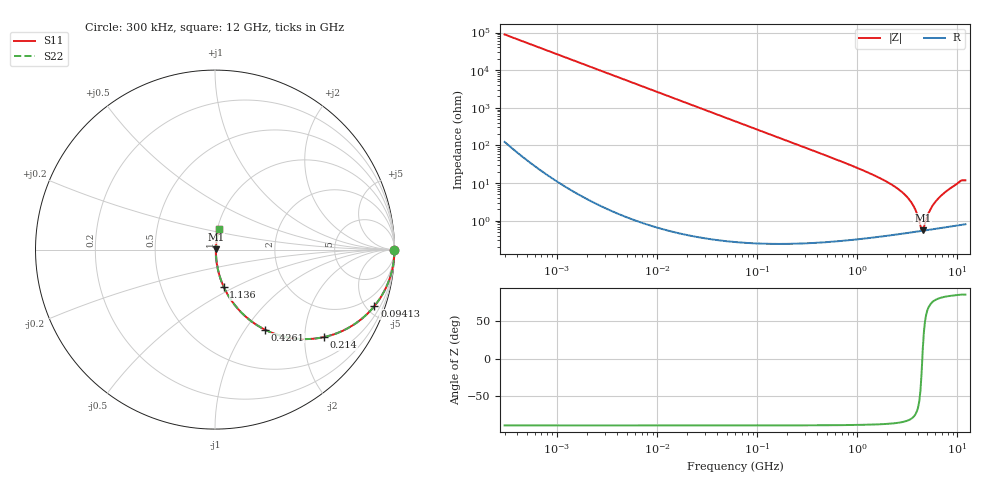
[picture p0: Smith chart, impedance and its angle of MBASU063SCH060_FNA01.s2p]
! MBASU063SCH060_FNA01  S-PARAMETER MODEL  ( Standard Model )
! Model Generated by TAIYO YUDEN Corporation (http://www.ty-top.com)
! Version 1.0
! TAIYO YUDEN Control No. 230609
! Copyright(c) 2023 TAIYO YUDEN CO.,LTD. All Rights Reserved.
! Product Description (link to TY-COMPAS)
! https://ds.yuden.co.jp/TYCOMPAS/or/detail?pn=MBASU063SCH060CFNA01&u=M
! Products Name : Multilayer Ceramic Capacitors
! Characteristics :
!  Capacitance : 6 [pF] , Rated Voltage : 50 [V] , TCC : CH / C0H
!  Case Size : 0.6 x 0.3 / 0.024 x 0.012 [mm/inch] , Thickness : 0.3 / 0.012 [mm/inch]
!  (Conditions: Temperature = 25 [degC] , DC Bias Voltage = 0 [V])
! External Node Assignments :
!  1  o---| |---o  2
! GND o---------o GND
! Frequency Range : 0.3MHz  -  12000MHz  [ 401 STEP ]
# MHZ S RI R 50
! Freq[MHz].  S11 Real  S11 Imag  S21 Real  S21 Imag  S12 Real  S12 Imag  S22 Real  S22 Imag
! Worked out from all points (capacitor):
!   401 points, 300 kHz to 12 GHz, reference 50 ohm
!   read as one part in series: C = 5.98 pF near 316.3 kHz
!   lowest |Z| = 557 mohm at 4.503 GHz (marker M1)
!   series resonance near 4.455 GHz, so ESL is about 210 pH
!   S11 on the Smith chart (normalised r, x): 300 kHz: open; 94.13 MHz: 1.01, -5.65; 214 MHz: 1.00, -2.48; 426.1 MHz: 1.01, -1.24; 1.136 GHz: 1.01, -0.44; 12 GHz: 1.02, +0.24
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0.3  1 -0.00113  2.85e-06 0.00113  2.85e-06 0.00113  1 -0.00113
1.769972  1 -0.00665  4.62e-05 0.00665  4.62e-05 0.00665  1 -0.00665
10.44266  0.9985 -0.0392  0.00155 0.0392  0.00155 0.0392  0.9985 -0.0392
27.82928  0.9891 -0.1035  0.0109 0.1035  0.0109 0.1035  0.9891 -0.1035
60  0.9515 -0.2146  0.0485 0.2146  0.0485 0.2146  0.9515 -0.2146
94.13233  0.8884 -0.3144  0.1116 0.3144  0.1116 0.3144  0.8884 -0.3144
213.9924  0.6058 -0.4877  0.3942 0.4877  0.3942 0.4877  0.6058 -0.4877
353.9943  0.3584 -0.4778  0.6416 0.4778  0.6416 0.4778  0.3584 -0.4778
426.1204  0.2776 -0.4457  0.7224 0.4457  0.7224 0.4457  0.2776 -0.4457
668.5285  0.1332 -0.3361  0.8668 0.3361  0.8668 0.3361  0.1332 -0.3361
1135.593  0.0486 -0.2077  0.9514 0.2077  0.9514 0.2077  0.0486 -0.2077
2088.533  0.0137 -0.0976  0.9863 0.0976  0.9863 0.0976  0.0137 -0.0976
2795.104  0.00777 -0.057  0.9922 0.057  0.9922 0.057  0.00777 -0.057
3364.605  0.00596 -0.0335  0.994 0.0335  0.994 0.0335  0.00596 -0.0335
3841.137  0.00538 -0.0175  0.9946 0.0175  0.9946 0.0175  0.00538 -0.0175
4270.516  0.00531 -0.00493  0.9947 0.00493  0.9947 0.00493  0.00531 -0.00493
4502.883  0.0054 0.00123  0.9946 -0.00123  0.9946 -0.00123  0.0054 0.00123
4623.766  0.00547 0.00396  0.9945 -0.00396  0.9945 -0.00396  0.00547 0.00396
5420.343  0.00621 0.0199  0.9938 -0.0199  0.9938 -0.0199  0.00621 0.0199
6354.153  0.00755 0.0367  0.9924 -0.0367  0.9924 -0.0367  0.00755 0.0367
10511.28  0.019 0.1058  0.981 -0.1058  0.981 -0.1058  0.019 0.1058
12000  0.0215 0.1149  0.9785 -0.1149  0.9785 -0.1149  0.0215 0.1149
